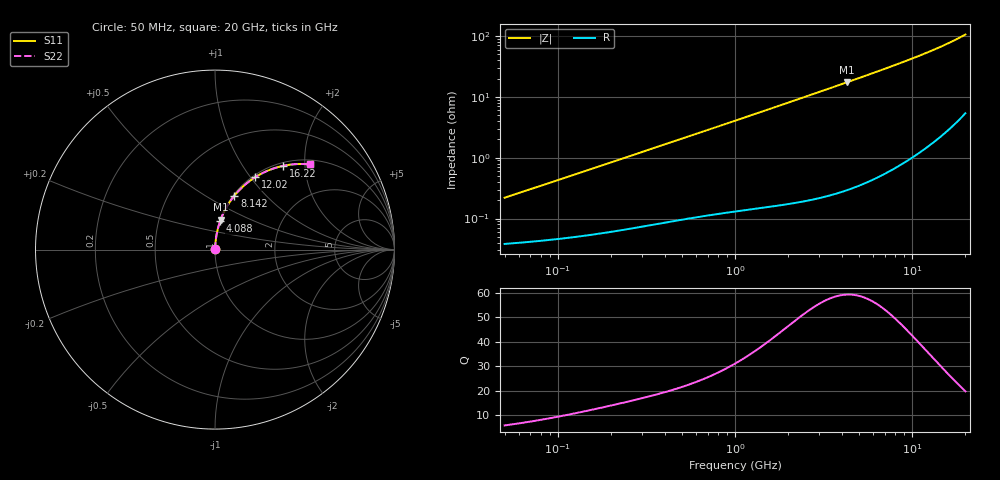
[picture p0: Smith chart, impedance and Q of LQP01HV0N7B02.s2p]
!Murata Part Number: LQP01HV0N7B02
!These Parameters are Measured in Series Mode Connection
!  o--[Z]--o
!Port1  Port2
!  o-------o
!Freq. Start=50[MHz] Stop=20[GHz], 401[Steps]
# Hz S RI R 50
!Freq.(Hz) S11(Real) S11(Imag) S21(Real) S21(Imag) S12(Real) S12(Imag) S22(Real) S22(Imag)
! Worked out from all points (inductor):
!   401 points, 50 MHz to 20 GHz, reference 50 ohm
!   read as one part in series: L = 685 pH near 51.52 MHz
!   highest Q = 59.4 at 4.276 GHz (marker M1), where L = 644 pH
!   S11 on the Smith chart (normalised r, x): 50 MHz: 1.00, +0.00; 4.088 GHz: 1.01, +0.33; 8.142 GHz: 1.01, +0.68; 12.02 GHz: 1.03, +1.05; 16.22 GHz: 1.06, +1.55; 20 GHz: 1.11, +2.12
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5e7  0.000387 0.00216  0.9996 -0.00216  0.9996 -0.00216  0.000387 0.00216
5.30873e7  0.000393 0.0023  0.9996 -0.0023  0.9996 -0.0023  0.000393 0.0023
1.364002e8  0.000547 0.00576  0.9995 -0.00576  0.9995 -0.00576  0.000547 0.00576
3.721004e8  0.00106 0.0153  0.9989 -0.0153  0.9989 -0.0153  0.00106 0.0153
6.380365e8  0.00175 0.0259  0.9983 -0.0259  0.9983 -0.0259  0.00175 0.0259
1e9  0.00293 0.0403  0.9971 -0.0403  0.9971 -0.0403  0.00293 0.0403
1.714689e9  0.00633 0.0685  0.9937 -0.0685  0.9937 -0.0685  0.00633 0.0685
2.728004e9  0.0139 0.108  0.9861 -0.108  0.9861 -0.108  0.0139 0.108
3.364474e9  0.0203 0.1326  0.9797 -0.1326  0.9797 -0.1326  0.0203 0.1326
4.087748e9  0.0291 0.16  0.9709 -0.16  0.9709 -0.16  0.0291 0.16
4.275624e9  0.0317 0.167  0.9683 -0.167  0.9683 -0.167  0.0317 0.167
5.769027e9  0.056 0.2214  0.944 -0.2214  0.944 -0.2214  0.056 0.2214
7.442007e9  0.0911 0.2783  0.9089 -0.2783  0.9089 -0.2783  0.0911 0.2783
8.141811e9  0.1081 0.3005  0.8919 -0.3005  0.8919 -0.3005  0.1081 0.3005
9.041845e9  0.1319 0.3277  0.8681 -0.3277  0.8681 -0.3277  0.1319 0.3277
1.004137e10  0.1606 0.3556  0.8394 -0.3556  0.8394 -0.3556  0.1606 0.3556
1.201863e10  0.2239 0.4033  0.7761 -0.4033  0.7761 -0.4033  0.2239 0.4033
1.396067e10  0.2928 0.4393  0.7072 -0.4393  0.7072 -0.4393  0.2928 0.4393
1.621653e10  0.3788 0.4664  0.6212 -0.4664  0.6212 -0.4664  0.3788 0.4664
1.800918e10  0.4494 0.4761  0.5506 -0.4761  0.5506 -0.4761  0.4494 0.4761
1.940974e10  0.5048 0.4763  0.4952 -0.4763  0.4952 -0.4763  0.5048 0.4763
2e10  0.528 0.4744  0.472 -0.4744  0.472 -0.4744  0.528 0.4744
